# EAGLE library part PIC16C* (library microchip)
MICROCONTROLLER PIC16C5X family: EPROM/ROM-based PIC16C55X family: EPROM-based PIC16C6X family PIC16CE62X family: analog comparators/EEPROM data memory PIC16C7X family: A/D converter PIC16C71X family: A/D converter PIC16F8X family: flash EEPROM Pin compatible devices: PIC16C154, PIC16CR154, PIC16C156, PIC16CR156, PIC16C158 PIC16CR158, PIC16C52, PIC16C54, PIC16C54A, PIC16CR54A PIC16C56, PIC16C58A, PIC16CR58A, PIC16C61, PIC16C554 PIC16C556, PIC16C558, PIC16C620, PIC16C621, PIC16C622 PIC16C641, PIC16C642, PIC16C661, PIC16C662, PIC16C71 PIC16C710, PIC16C711, PIC16C715, PIC126F83, PIC16CR83 PIC16F84A, PIC16CR84 see also PIC16F8*
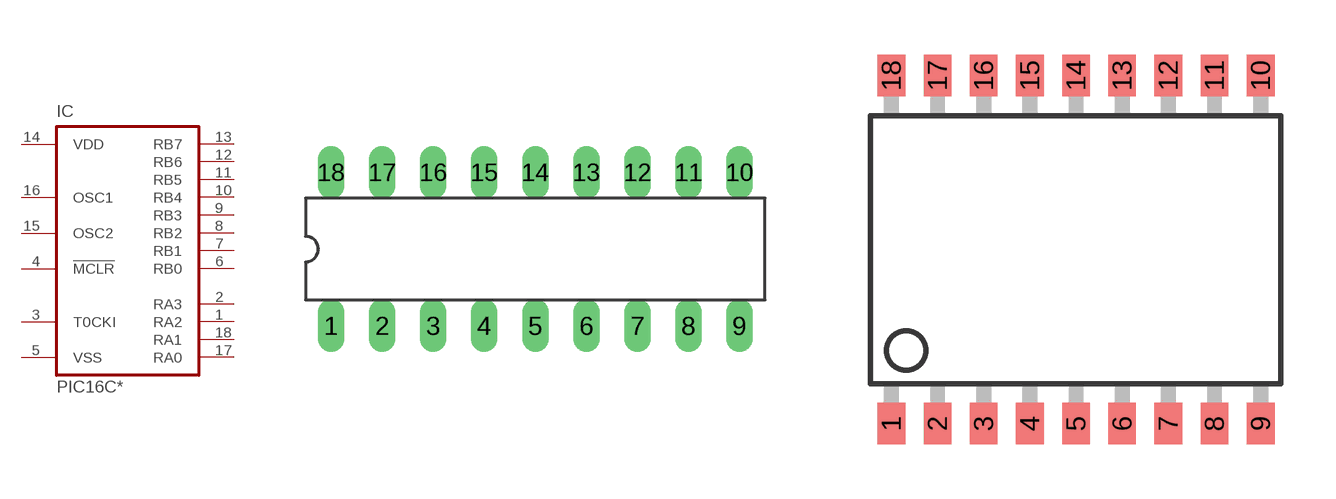
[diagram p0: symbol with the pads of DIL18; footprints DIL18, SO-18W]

Designator prefix IC

## PIC16C154P (OC_FARNELL: unknown; OC_NEWARK: unknown), PIC16C156P (OC_FARNELL: unknown; OC_NEWARK: unknown), PIC16C158P (OC_FARNELL: unknown; OC_NEWARK: unknown), PIC16C52P (OC_FARNELL: unknown; OC_NEWARK: unknown), PIC16C54P (MF: MICROCHIP; MPN: PIC16C54-RCI/P; OC_FARNELL: 1084285; OC_NEWARK: 23C3204), PIC16C54AP (MF: MICROCHIP; MPN: PIC16C54A-04/P; OC_FARNELL: 1196847; OC_NEWARK: 61K3438), PIC16C55P (MF: MICROCHIP; MPN: PIC16C558-04/P; OC_FARNELL: 1084353; OC_NEWARK: 96K3797), PIC16C554P (MF: MICROCHIP; MPN: PIC16C554-04I/P; OC_FARNELL: 9759204; OC_NEWARK: 23C3455), PIC16C556P (OC_FARNELL: unknown; OC_NEWARK: unknown), PIC16C558P (MPN: PIC16C558-20/P; OC_FARNELL: 9759220; OC_NEWARK: 97K7200), PIC16C56P (MF: MICROCHIP; MPN: PIC16C56-HS/P; OC_FARNELL: 1084307; OC_NEWARK: 23C3511), PIC16C58AP (MF: MICROCHIP; MPN: PIC16C58B-04/P; OC_FARNELL: 9759417; OC_NEWARK: 23C3736), PIC16C61P (OC_FARNELL: unknown; OC_NEWARK: unknown), PIC16C620P (MPN: PIC16C620-04/P; OC_FARNELL: 1196828; OC_NEWARK: 24M5866), PIC16C621P (MF: MICROCHIP; MPN: PIC16C621-04I/P; OC_FARNELL: 1196829; OC_NEWARK: 23C3904), PIC16C622P (MF: MICROCHIP; MPN: PIC16C622A-04I/P; OC_FARNELL: 9759549; OC_NEWARK: 23C3984), PIC16C641P (OC_FARNELL: unknown; OC_NEWARK: unknown), PIC16C661P (OC_FARNELL: unknown; OC_NEWARK: unknown), PIC16C71P (MF: MICROCHIP; MPN: PIC16C71-20I/P; OC_FARNELL: 1196825; OC_NEWARK: 73K1290), PIC16C710P (MF: MICROCHIP; MPN: PIC16C71-04/P; OC_FARNELL: 9759778; OC_NEWARK: 69K7626), PIC16C711P (MF: MICROCHIP; MPN: PIC16C711-04I/P; OC_FARNELL: 1084359; OC_NEWARK: 68K5331), PIC16C715P (MPN: PIC16C715-20/P; OC_FARNELL: 1084360; OC_NEWARK: 97K7271), PIC16C84P (OC_FARNELL: unknown; OC_NEWARK: unknown), PIC16CF83P (OC_FARNELL: unknown; OC_NEWARK: unknown), PIC16CR154P (OC_FARNELL: unknown; OC_NEWARK: unknown), PIC16CR156P (OC_FARNELL: unknown; OC_NEWARK: unknown), PIC16CR158P (OC_FARNELL: unknown; OC_NEWARK: unknown), PIC16CR54P (OC_FARNELL: unknown; OC_NEWARK: unknown), PIC16CR54AP (OC_FARNELL: unknown; OC_NEWARK: unknown), PIC16CR58AP (OC_FARNELL: unknown; OC_NEWARK: unknown), PIC16CR83P (OC_FARNELL: unknown; OC_NEWARK: unknown), PIC16CR84P (OC_FARNELL: unknown; OC_NEWARK: unknown)  [DIL18]
1  RA2
2  RA3
3  T0CKI  in
4  !MCLR  in
5  VSS  pwr
6  RB0
7  RB1
8  RB2
9  RB3
10  RB4
11  RB5
12  RB6
13  RB7
14  VDD  pwr
15  OSC2  out
16  OSC1  in
17  RA0
18  RA1

## PIC16C154SO (OC_FARNELL: unknown; OC_NEWARK: unknown), PIC16C156SO (OC_FARNELL: unknown; OC_NEWARK: unknown), PIC16C158SO (OC_FARNELL: unknown; OC_NEWARK: unknown), PIC16C52SO (OC_FARNELL: unknown; OC_NEWARK: unknown), PIC16C54SO (MF: MICROCHIP; MPN: PIC16C54-XT/SO; OC_FARNELL: 9759182; OC_NEWARK: 23C3207), PIC16C54ASO (MF: MICROCHIP; MPN: PIC16C54A-04I/SO; OC_FARNELL: 1084342; OC_NEWARK: 23C3231), PIC16C55SO (OC_FARNELL: unknown; OC_NEWARK: unknown), PIC16C554SO (MPN: PIC16C554-04/SO; OC_FARNELL: 1084352; OC_NEWARK: 97K7196), PIC16C556SO (OC_FARNELL: unknown; OC_NEWARK: unknown), PIC16C558SO (MF: MICROCHIP; MPN: PIC16C558-04/SO; OC_FARNELL: unknown; OC_NEWARK: 23C3481), PIC16C58ASO (OC_FARNELL: unknown; OC_NEWARK: unknown), PIC16C61SO (OC_FARNELL: unknown; OC_NEWARK: unknown), PIC16C620SO (MF: MICROCHIP; MPN: PIC16C620-04/SO; OC_FARNELL: 9759468; OC_NEWARK: 23C3838), PIC16C621SO (MF: MICROCHIP; MPN: PIC16C621-04I/SO; OC_FARNELL: 9759492; OC_NEWARK: 23C3905), PIC16C622SO (MF: MICROCHIP; MPN: PIC16C622A-04I/SO; OC_FARNELL: 9759522; OC_NEWARK: 23C3985), PIC16C71SO (OC_FARNELL: unknown; OC_NEWARK: unknown), PIC16C710SO (MF: MICROCHIP; MPN: PIC16C710-20/SO; OC_FARNELL: unknown; OC_NEWARK: 23C4447), PIC16C711SO (MF: MICROCHIP; MPN: PIC16C711-20/SO; OC_FARNELL: 9759808; OC_NEWARK: 12C1918), PIC16C715SO (MF: MICROCHIP; MPN: PIC16C715-04I/SO; OC_FARNELL: 1084362; OC_NEWARK: 23C4530), PIC16C84SO (OC_FARNELL: unknown; OC_NEWARK: unknown), PIC16CR154SO (OC_FARNELL: unknown; OC_NEWARK: unknown), PIC16CR156SO (OC_FARNELL: unknown; OC_NEWARK: unknown), PIC16CR158SO (OC_FARNELL: unknown; OC_NEWARK: unknown), PIC16CR54SO (OC_FARNELL: unknown; OC_NEWARK: unknown), PIC16CR54ASO (OC_FARNELL: unknown; OC_NEWARK: unknown), PIC16CR58ASO (OC_FARNELL: unknown; OC_NEWARK: unknown), PIC16CR83SO (OC_FARNELL: unknown; OC_NEWARK: unknown), PIC16CR84SO (OC_FARNELL: unknown; OC_NEWARK: unknown)  [SO-18W]
Pads as for DIL18

## Footprint DIL18 (pad centres in mm)
Dual In Line package type P
drill 0.813 long: 1 -10.16,-3.81; 2 -7.62,-3.81; 3 -5.08,-3.81; 4 -2.54,-3.81; 5 0,-3.81; 6 2.54,-3.81; 7 5.08,-3.81; 8 7.62,-3.81; 9 10.16,-3.81; 10 10.16,3.81; 11 7.62,3.81; 12 5.08,3.81; 13 2.54,3.81; 14 0,3.81; 15 -2.54,3.81; 16 -5.08,3.81; 17 -7.62,3.81; 18 -10.16,3.81

## Footprint SO-18W (pad centres in mm)
Small Outline Wide Plastic Gull Wing 300-mil body, package type SO
smd 0.762 x 1.143: 1 -5.08,-4.788; 2 -3.81,-4.788; 3 -2.54,-4.788; 4 -1.27,-4.788; 5 0,-4.788; 6 1.27,-4.788; 7 2.54,-4.788; 8 3.81,-4.788; 9 5.08,-4.788; 10 5.08,4.788; 11 3.81,4.788; 12 2.54,4.788; 13 1.27,4.788; 14 0,4.788; 15 -1.27,4.788; 16 -2.54,4.788; 17 -3.81,4.788; 18 -5.08,4.788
